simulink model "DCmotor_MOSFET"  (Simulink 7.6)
settings: Solver=ode23tb  StartTime=0.0  StopTime=10  RelTol=1e-3
StopFcn:
  | close all
  | load DCMotor_MOSFET.mat
  | subplot 211
  | plot(x(1,:),x(2,:))
  | grid
  | title('Vitesse du moteur et couple résistant')
  | axis([0 10 -20 200])
  | hold on
  | plot(x(1,:),x(3,:))
  | subplot 212
  | plot(x(1,:),x(4,:))
  | grid
  | axis([0 10 -0.2 1.2])
  | title('Commande de la gachette')
  | xlabel('temps')
  | % axis([0 2 -.2 1.2])
  | delete *.mat
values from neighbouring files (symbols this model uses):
  A = [1+j -(1-j);1 -2/(1-j)]    [systeme_AX_B_phaseurs.m]
  N = 50;')    [Prog_callbacks.m]    (also in _startup.m = 0.001'))
undefined symbols (not defined in the file or in its folder): constant, Torque
libraries: powerlib x7

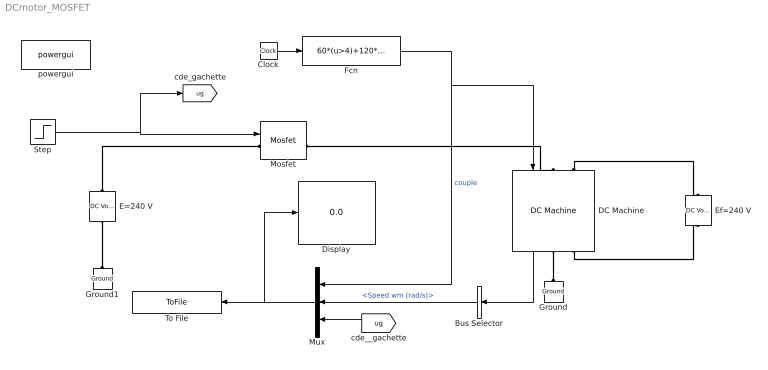
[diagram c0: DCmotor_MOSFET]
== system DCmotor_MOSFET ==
  Bus Selector : BusSelector  OutputSignals=Speed wm (rad/s)
  Clock : Clock
  DC Machine : powerlib/Machines/DC Machine  DialogController=POWERSYS.PowerSysDialog  SystemSampleTime=-1  PresetModel=No  MechanicalLoad=Torque TL  FieldType=Wound  ShowDetailedParameters=on  RLa="[ 0.6  0.012]"  RLf="[ 240  120]"  Laf=1.8  MachineConstant=Torque constant (N.m/A)  Ke=1.8  Kt=1.8  J=1  Bm=0  Tf=0  w0=1  Ifinit=1  TsPowergui=0  TsBlock=-1
  Display : Display
  E=240 V : powerlib/Electrical Sources/DC Voltage Source  Description=source block  DialogController=POWERSYS.PowerSysDialog  SystemSampleTime=-1  Amplitude=240  Measurements=None
  Ef=240 V : powerlib/Electrical Sources/DC Voltage Source  Description=source block  DialogController=POWERSYS.PowerSysDialog  SystemSampleTime=-1  Amplitude=240  Measurements=None
  Fcn : Fcn  Expr=60*(u>4)+120*(u>6)
  Ground : powerlib/Elements/Ground  DialogController=POWERSYS.PowerSysDialog  PhysicalDomain=powersysdomain  SubClassName=unknown  LeftPortType=p1  RightPortType=p1  LConnTagsString=a
  Ground1 : powerlib/Elements/Ground  DialogController=POWERSYS.PowerSysDialog  PhysicalDomain=powersysdomain  SubClassName=unknown  LeftPortType=p1  RightPortType=p1  LConnTagsString=a
  Mosfet : powerlib/Power Electronics/Mosfet  DialogController=POWERSYS.PowerSysDialog  SystemSampleTime=-1  Ron=0.1  Lon=0  Rd=0.01  Vfd=0  IC=0  Rs=1e5  Cs=inf  Measurements=on
  Mux : Mux  Inputs=3
  Step : Step  SampleTime=0
  To File : ToFile  Filename=DCMotor_MOSFET  MatrixName=x
  powergui : powerlib/powergui  SystemSampleTime=-1  SimulationMode=Continuous  SampleTime=5e-9  frequency=60  SPID=off  DisableSnubberDevices=off  DisableRonSwitches=off  DisableVfSwitches=off  SwTol=0  Interpol=off  frequencyindice=0  echomessages=off  HookPort=off  DisplayEquations=off  FunctionMessages=off  EnableUseOfTLC=off  x0status=blocks  RestoreLinks=warning  ResistiveCurrentMeasurement=off  Frange=[0:2:500]  Ylog=off  Xlog=on  ShowGrid=off  save=off  variable=ZData  ZoomFFT=on  StartTime=0.0  cycles=1  DisplayStyle=1  fundamental=60  FreqAxis=off  MaxFrequency=1000  frequencyindicesteady=1  RmsSteady=1  display=off  Ts=0  methode=off
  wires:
  Fcn/1 -> DC Machine/1, Mux/1  "couple"
  Step/1 -> Mosfet/1, [ug]
  Mux/1 -> To File/1, Display/1
  DC Machine/1 -> Bus Selector/1
  Bus Selector/1 -> Mux/2  "<Speed wm (rad/s)>"
  Clock/1 -> Fcn/1
  [ug] -> Mux/3
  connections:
  DC Machine/RConn1 -- Ground/LConn1
  E=240 V/LConn1 -- Ground1/LConn1
  DC Machine/LConn2 -- Ef=240 V/RConn1
  DC Machine/RConn2 -- Ef=240 V/LConn1
  E=240 V/RConn1 -- Mosfet/LConn1
  Mosfet/RConn1 -- DC Machine/LConn1
